FUNCTION "FC_BASIC FUNCTIONS" : VOID
TITLE =BASIC FUNCTIONS
VERSION : 0.1


VAR_TEMP
  DUMMY_BOOL : BOOL ;
  DUMMY_INT : INT ;
END_VAR
BEGIN
NETWORK
TITLE =LOGICAL "0" AND "1"
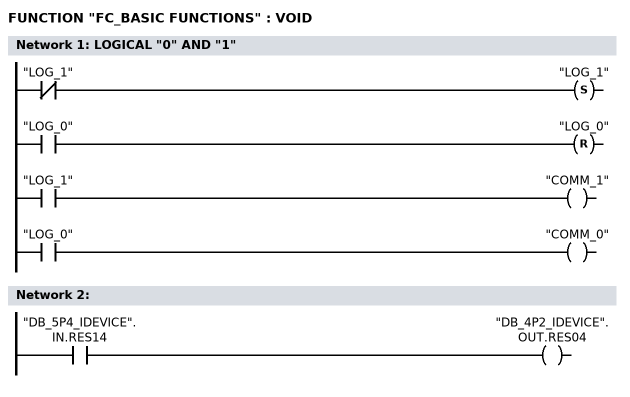
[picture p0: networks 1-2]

      UN    "LOG_1";
      S     "LOG_1";


      U     "LOG_0";
      R     "LOG_0";


      U     "LOG_1";
      =     "COMM_1";

      U     "LOG_0";
      =     "COMM_0";
NETWORK
TITLE =

      U     "DB_5P4_IDEVICE".IN.RES14;
      =     "DB_4P2_IDEVICE".OUT.RES04;
NETWORK
TITLE =EDGES AND TACT MARKERS

      L     "MB_CLOCKBYTE";
      L     "MB_EDGE_MARKER";
      XOW   ;
      UW    ;
      T     "MB_IMPULSE_MARKER";
      L     "MB_CLOCKBYTE";
      T     "MB_EDGE_MARKER";

NETWORK
TITLE =PULSE EVERY 1 SECOND m2.5

NETWORK
TITLE =DELAY ON TIME - RELEASE TO START MOTORS 15 SECONDS

      U(    ;
      U     "DELAY_ON_15s";
      UN    "DELAY_ON_15s_mem";
      L     S5T#15S;
      SE    "T_DELAY_15s";
      NOP   0;
      NOP   0;
      NOP   0;
      U     "T_DELAY_15s";
      )     ;
      =     "DELAY_ON_15s_mem";
      U     "DELAY_ON_15s_mem";
      R     "DELAY_ON_15s";
NETWORK
TITLE =DELAY ON TIME - RELEASE TO START MOTORS 0 SECONDS

      U     "DELAY_ON_0s";
      R     "DELAY_ON_0s";
NETWORK
TITLE =DELAY ON TIME - RELEASE TO START MOTORS 30 SECONDS

      U(    ;
      U     "DELAY_ON_OVEN";
      UN    "DELAY_ON_OVEN_mem";
      L     S5T#30S;
      SE    "T_DELAY_OVEN";
      NOP   0;
      NOP   0;
      NOP   0;
      U     "T_DELAY_OVEN";
      )     ;
      =     "DELAY_ON_OVEN_mem";
      U     "DELAY_ON_OVEN_mem";
      R     "DELAY_ON_OVEN";
NETWORK
TITLE =********* PULSE FOR FLAP OF BURNER *****************

NETWORK
TITLE =PULSE 2S, 15S PAUSE
//Was change from 15s to 1min for test
//19.04.2016 - VT
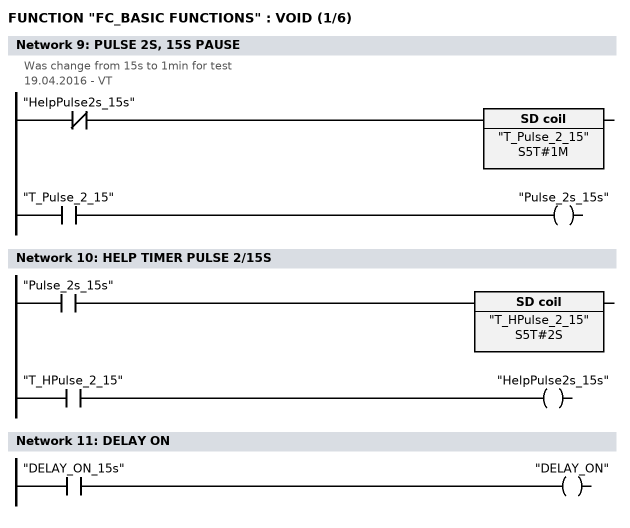
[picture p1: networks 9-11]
      UN    "HelpPulse2s_15s";
      L     S5T#1M;
      SE    "T_Pulse_2_15";
      NOP   0;
      NOP   0;
      NOP   0;
      U     "T_Pulse_2_15";
      =     "Pulse_2s_15s";
NETWORK
TITLE =HELP TIMER PULSE 2/15S

      U     "Pulse_2s_15s";
      L     S5T#2S;
      SE    "T_HPulse_2_15";
      NOP   0;
      NOP   0;
      NOP   0;
      U     "T_HPulse_2_15";
      =     "HelpPulse2s_15s";
NETWORK
TITLE =DELAY ON

      U     "DELAY_ON_15s";
      =     "DELAY_ON";
NETWORK
TITLE =MASTER RESET OVEN/WORKDECKS
//
//********************** MASTER/OVEN/WORKDECKS RESET *****************************
//
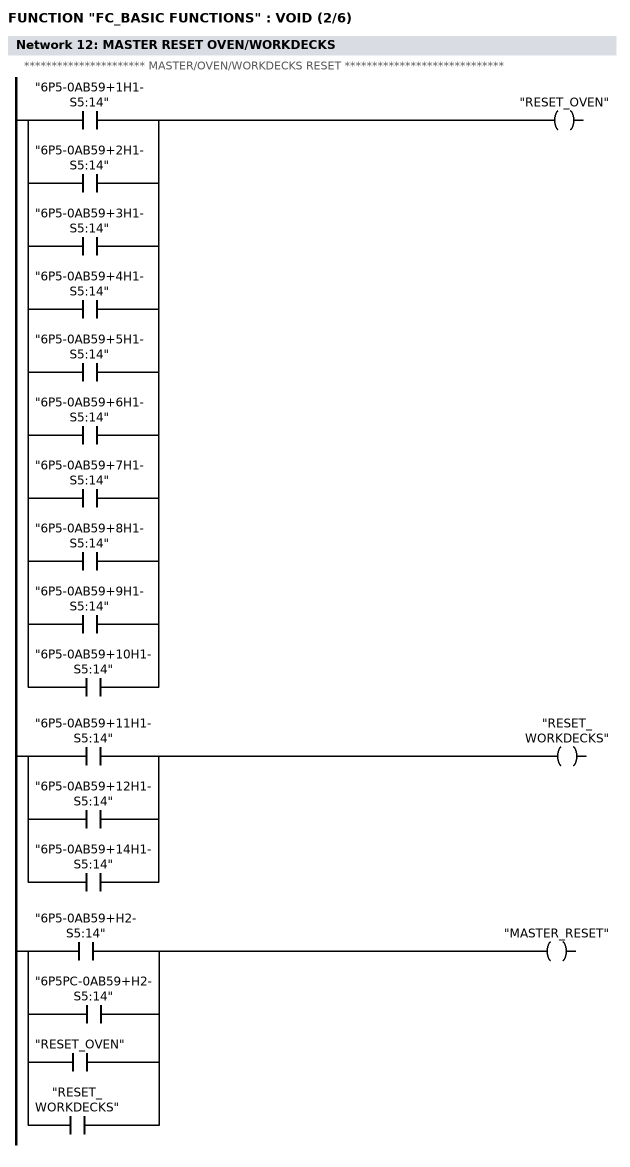
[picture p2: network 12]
      U     "6P5-0AB59+1H1-S5:14";
      O     "6P5-0AB59+2H1-S5:14";
      O     "6P5-0AB59+3H1-S5:14";
      O     "6P5-0AB59+4H1-S5:14";
      O     "6P5-0AB59+5H1-S5:14";
      O     "6P5-0AB59+6H1-S5:14";
      O     "6P5-0AB59+7H1-S5:14";
      O     "6P5-0AB59+8H1-S5:14";
      O     "6P5-0AB59+9H1-S5:14";
      O     "6P5-0AB59+10H1-S5:14";
      =     "RESET_OVEN";

      U     "6P5-0AB59+11H1-S5:14";
      O     "6P5-0AB59+12H1-S5:14";
      O     "6P5-0AB59+14H1-S5:14";
      =     "RESET_WORKDECKS";


      U     "6P5-0AB59+H2-S5:14";
      O     "6P5PC-0AB59+H2-S5:14";
      O     "RESET_OVEN";
      O     "RESET_WORKDECKS";
      =     "MASTER_RESET";


NETWORK
TITLE =MASTER RESET SIREN OVEN/WORKDECKS
//
//******************** MASTER/OVEN/WORKDECKS RESET SIREN **********************
//
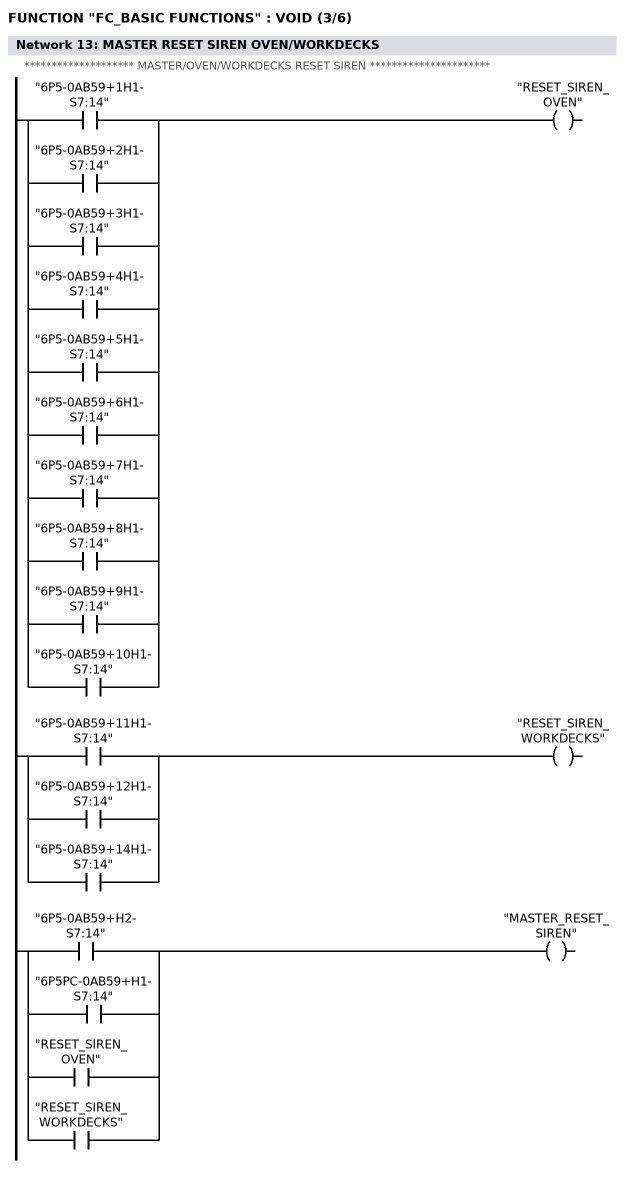
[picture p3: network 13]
      U     "6P5-0AB59+1H1-S7:14";
      O     "6P5-0AB59+2H1-S7:14";
      O     "6P5-0AB59+3H1-S7:14";
      O     "6P5-0AB59+4H1-S7:14";
      O     "6P5-0AB59+5H1-S7:14";
      O     "6P5-0AB59+6H1-S7:14";
      O     "6P5-0AB59+7H1-S7:14";
      O     "6P5-0AB59+8H1-S7:14";
      O     "6P5-0AB59+9H1-S7:14";
      O     "6P5-0AB59+10H1-S7:14";
      =     "RESET_SIREN_OVEN";

      U     "6P5-0AB59+11H1-S7:14";
      O     "6P5-0AB59+12H1-S7:14";
      O     "6P5-0AB59+14H1-S7:14";
      =     "RESET_SIREN_WORKDECKS";


      U     "6P5-0AB59+H2-S7:14";
      O     "6P5PC-0AB59+H1-S7:14";
      O     "RESET_SIREN_OVEN";
      O     "RESET_SIREN_WORKDECKS";
      =     "MASTER_RESET_SIREN";


NETWORK
TITLE =IS ERROR OVEN/WORKDECKS
//
//********************** IS ERROR OVEN/WORKDECKS **********************
//
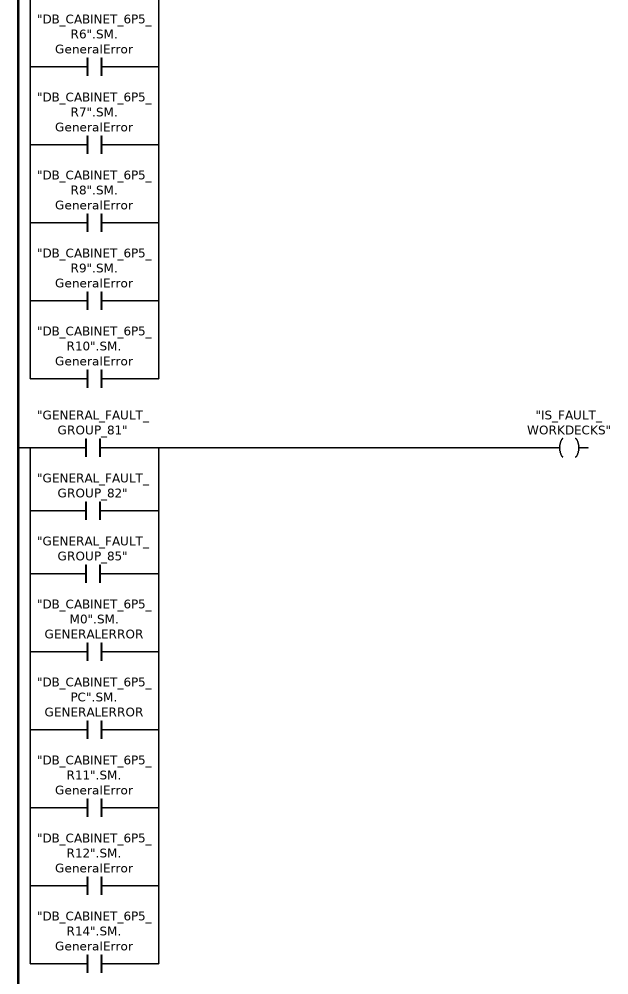
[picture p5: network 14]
      U     "GENERAL_FAULT_GROUP_00";
      O     "GENERAL_FAULT_GROUP_01";
      O     "GENERAL_FAULT_GROUP_02";
      O     "GENERAL_FAULT_GROUP_03";
      O     "GENERAL_FAULT_GROUP_04";
      O     "GENERAL_FAULT_GROUP_11";
      O     "GENERAL_FAULT_GROUP_12";
      O     "GENERAL_FAULT_GROUP_15";
      O     "GENERAL_FAULT_GROUP_20";
      O     "GENERAL_FAULT_GROUP_21";
      O     "GENERAL_FAULT_GROUP_30";
      O     "GENERAL_FAULT_GROUP_31";
      O     "DB_CABINET_6P5_M0".SM.GENERALERROR;
      O     "DB_CABINET_6P5_PC".SM.GENERALERROR;
      O     "DB_CABINET_6P5_R1".SM.GeneralError;
      O     "DB_CABINET_6P5_R2".SM.GeneralError;
      O     "DB_CABINET_6P5_R3".SM.GeneralError;
      O     "DB_CABINET_6P5_R4".SM.GeneralError;
      O     "DB_CABINET_6P5_R5".SM.GeneralError;
      O     "DB_CABINET_6P5_R6".SM.GeneralError;
      O     "DB_CABINET_6P5_R7".SM.GeneralError;
      O     "DB_CABINET_6P5_R8".SM.GeneralError;
      O     "DB_CABINET_6P5_R9".SM.GeneralError;
      O     "DB_CABINET_6P5_R10".SM.GeneralError;
      =     "IS_FAULT_OVEN";

      U     "GENERAL_FAULT_GROUP_81";
      O     "GENERAL_FAULT_GROUP_82";
      O     "GENERAL_FAULT_GROUP_85";
      O     "DB_CABINET_6P5_M0".SM.GENERALERROR;
      O     "DB_CABINET_6P5_PC".SM.GENERALERROR;
      O     "DB_CABINET_6P5_R11".SM.GeneralError;
      O     "DB_CABINET_6P5_R12".SM.GeneralError;
      O     "DB_CABINET_6P5_R14".SM.GeneralError;
      =     "IS_FAULT_WORKDECKS";



NETWORK
TITLE =WAS MANUAL MODE ON THE CABINET (FOR VISU)
//
//********************** WAS MANUAL MODE LINE_1/LINE_2 **********************
//
// OVEN
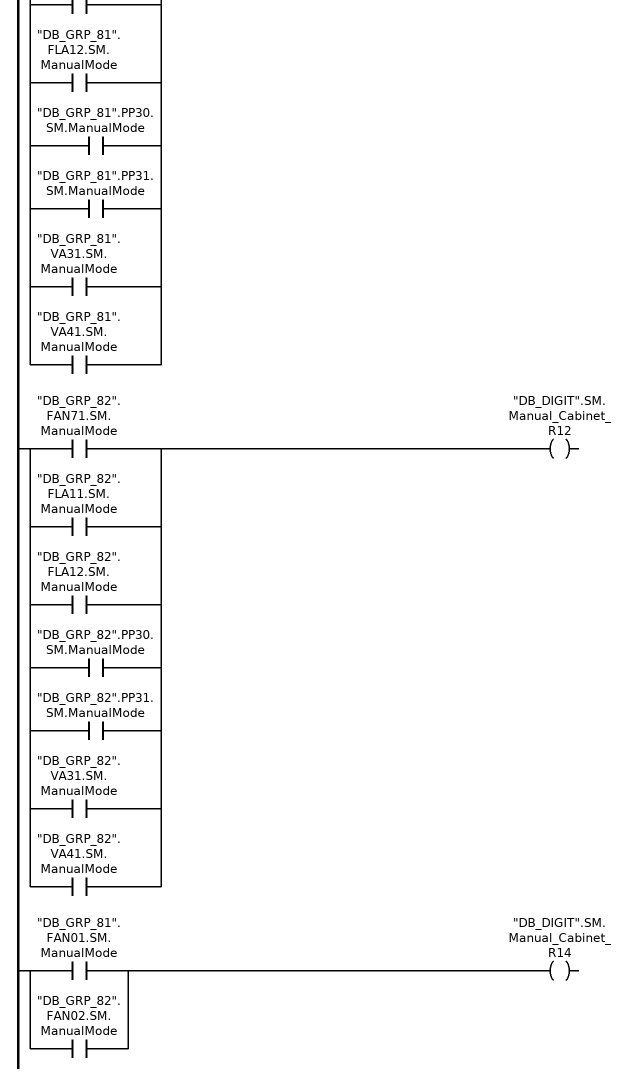
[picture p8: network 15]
      U     "DB_GRP_01".FAN01_M1.SM.ManualMode;
      O     "DB_GRP_01".FLA02_M1.SM.ManualMode;
      =     "DB_DIGIT".SM.Manual_Cabinet_R1;

      U     "DB_GRP_02".FAN01_M1.SM.ManualMode;
      O     "DB_GRP_02".FLA02_M1.SM.ManualMode;
      =     "DB_DIGIT".SM.Manual_Cabinet_R2;

      U     "DB_GRP_03".FAN01_M1.SM.ManualMode;
      O     "DB_GRP_03".FLA02_M1.SM.ManualMode;
      =     "DB_DIGIT".SM.Manual_Cabinet_R3;

      U     "DB_GRP_04".FAN01_M1.SM.ManualMode;
      O     "DB_GRP_04".FLA02_M1.SM.ManualMode;
      =     "DB_DIGIT".SM.Manual_Cabinet_R4;

      U     "DB_GRP_11".FAN01_M1.SM.ManualMode;
      O     "DB_GRP_11".FLA02_M1.SM.ManualMode;
      =     "DB_DIGIT".SM.Manual_Cabinet_R5;

      U     "DB_GRP_12".FAN01_M1.SM.ManualMode;
      O     "DB_GRP_12".FLA02_M1.SM.ManualMode;
      =     "DB_DIGIT".SM.Manual_Cabinet_R6;

      U     "DB_GRP_15".FAN01_M1.SM.ManualMode;
      O     "DB_GRP_15".FLA02_M1.SM.ManualMode;
      =     "DB_DIGIT".SM.Manual_Cabinet_R7;

      U     "DB_GRP_20".FAN01.SM.ManualMode;
      =     "DB_DIGIT".SM.Manual_Cabinet_R8;


      U     "DB_GRP_30".FAN01_M1.SM.ManualMode;
      O     "DB_GRP_30".FLA02_Y1.SM.ManualMode;
      O     "DB_GRP_30".FLA03_Y1.SM.ManualMode;
      O     "DB_GRP_30".PP10_M1.SM.ManualMode;
      O     "DB_GRP_30".VA11_M1.SM.ManualMode;
      O     "DB_GRP_31".FAN01.SM.ManualMode;
      O     "DB_GRP_31".FAN03.SM.ManualMode;
      O     "DB_GRP_31".FAN31.SM.ManualMode;
      O     "DB_GRP_31".FLA02.SM.ManualMode;
      O     "DB_GRP_31".FLA12_M1.SM.ManualMode;
      O     "DB_GRP_31".FLA12_M2.SM.ManualMode;
      O     "DB_GRP_31".VA21.SM.ManualMode;
      O     "DB_GRP_85".FAN94.SM.ManualMode;
      O     "DB_GRP_85".FLA95_M1.SM.ManualMode;
      O     "DB_GRP_85".TAN01_Y10.SM.ManualMode;
      =     "DB_DIGIT".SM.Manual_Cabinet_R9;

      U     "DB_GRP_21".FLA01.SM.ManualMode;
      O     "DB_GRP_21".CAS01.SM.ManualMode;
      =     "DB_DIGIT".SM.Manual_Cabinet_R10;

// WORKDECKS
      U     "DB_GRP_81".FAN71.SM.ManualMode;
      O     "DB_GRP_81".FLA11.SM.ManualMode;
      O     "DB_GRP_81".FLA12.SM.ManualMode;
      O     "DB_GRP_81".PP30.SM.ManualMode;
      O     "DB_GRP_81".PP31.SM.ManualMode;
      O     "DB_GRP_81".VA31.SM.ManualMode;
      O     "DB_GRP_81".VA41.SM.ManualMode;
      =     "DB_DIGIT".SM.Manual_Cabinet_R11;

      U     "DB_GRP_82".FAN71.SM.ManualMode;
      O     "DB_GRP_82".FLA11.SM.ManualMode;
      O     "DB_GRP_82".FLA12.SM.ManualMode;
      O     "DB_GRP_82".PP30.SM.ManualMode;
      O     "DB_GRP_82".PP31.SM.ManualMode;
      O     "DB_GRP_82".VA31.SM.ManualMode;
      O     "DB_GRP_82".VA41.SM.ManualMode;
      =     "DB_DIGIT".SM.Manual_Cabinet_R12;

      U     "DB_GRP_81".FAN01.SM.ManualMode;
      O     "DB_GRP_82".FAN02.SM.ManualMode;
      =     "DB_DIGIT".SM.Manual_Cabinet_R14;




NETWORK
TITLE =DUMMY FUNCTION
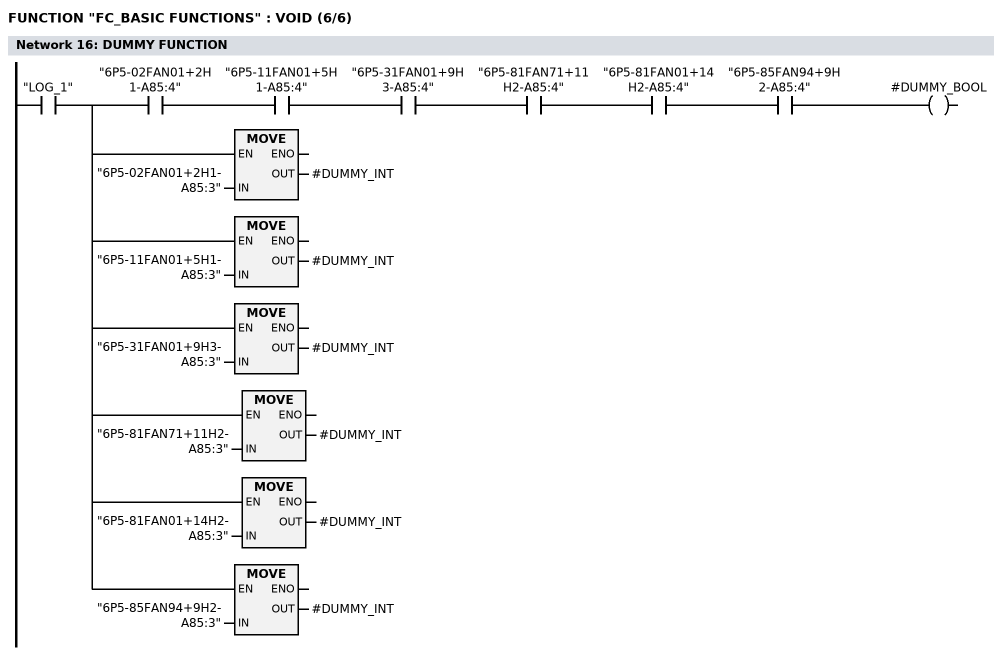
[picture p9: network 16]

      U     "LOG_1";
      =     L      4.0;
      U     L      4.0;
      U     "6P5-02FAN01+2H1-A85:4";
      U     "6P5-11FAN01+5H1-A85:4";
      U     "6P5-31FAN01+9H3-A85:4";
      U     "6P5-81FAN71+11H2-A85:4";
      U     "6P5-81FAN01+14H2-A85:4";
      U     "6P5-85FAN94+9H2-A85:4";
      =     #DUMMY_BOOL;
      U     L      4.0;
      SPBNB _001;
      L     "6P5-02FAN01+2H1-A85:3";
      T     #DUMMY_INT;
_001: NOP   0;
      U     L      4.0;
      SPBNB _002;
      L     "6P5-11FAN01+5H1-A85:3";
      T     #DUMMY_INT;
_002: NOP   0;
      U     L      4.0;
      SPBNB _003;
      L     "6P5-31FAN01+9H3-A85:3";
      T     #DUMMY_INT;
_003: NOP   0;
      U     L      4.0;
      SPBNB _004;
      L     "6P5-81FAN71+11H2-A85:3";
      T     #DUMMY_INT;
_004: NOP   0;
      U     L      4.0;
      SPBNB _005;
      L     "6P5-81FAN01+14H2-A85:3";
      T     #DUMMY_INT;
_005: NOP   0;
      U     L      4.0;
      SPBNB _006;
      L     "6P5-85FAN94+9H2-A85:3";
      T     #DUMMY_INT;
_006: NOP   0;
NETWORK
TITLE =END

END_FUNCTION

